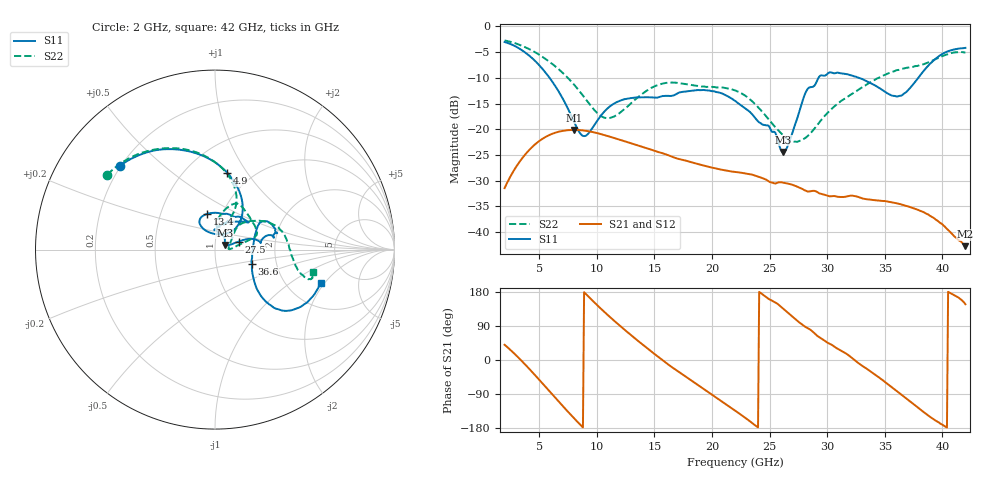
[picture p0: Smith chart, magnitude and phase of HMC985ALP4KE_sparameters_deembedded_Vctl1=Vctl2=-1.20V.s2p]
!s2p File: Measurements: S11, S21, S12, S22
# GHz S dB R 50.0
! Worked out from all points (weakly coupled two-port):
!   401 points, 2 GHz to 42 GHz, reference 50 ohm
!   highest |S21| = -20.11 dB at 8 GHz (marker M1); lowest = -42.7 dB at 42 GHz (marker M2)
!   lowest |S11| = -24.4 dB at 26.2 GHz (marker M3), VSWR 1.13, Z = 55.7 + j2.87 ohm
!   |S11| at or under -10 dB: 5.908 GHz to 29.25 GHz (23.34 GHz wide, 133 % of centre); 32.76 GHz to 37.9 GHz (5.142 GHz wide, 14.6 % of centre)
!   |S22| runs from -22.4 to -2.7 dB; largest |S21 - S12| = 0.00014
!   S11 on the Smith chart (normalised r, x): 2 GHz: 0.20, +0.37; 4.9 GHz: 0.77, +0.81; 13.4 GHz: 0.85, +0.35; 27.5 GHz: 1.30, +0.12; 36.6 GHz: 1.49, -0.25; 42 GHz: 3.03, -1.85
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2  -3.01 138.6  -31.43 40.1  -31.43 40.1  -2.72 145.2
3.4  -4.46 111.1  -26.00 0.2  -26.00 0.2  -3.66 122.3
4.9  -7.28 80.8  -22.44 -48.7  -22.45 -48.7  -5.34 98.8
6.2  -10.92 57.1  -20.81 -93.0  -20.82 -93.0  -7.39 80.8
8  -18.39 51.2  -20.11 -152.8  -20.11 -152.8  -11.23 64.7
8.7  -21.14 73.6  -20.19 -174.9  -20.19 -174.9  -13.15 63.4
10.9  -16.00 120.8  -21.27 120.2  -21.27 120.1  -17.82 81.9
13.4  -13.81 102.5  -23.01 54.9  -23.02 54.9  -14.09 80.9
15.4  -13.73 75.7  -24.45 7.0  -24.45 7.0  -11.30 68.5
18.9  -12.38 40.0  -26.81 -68.6  -26.82 -68.6  -11.60 41.8
22  -14.45 55.3  -28.27 -133.3  -28.28 -133.3  -12.43 18.4
24.9  -19.28 88.1  -30.06 161.6  -30.07 161.5  -18.01 10.1
26.2  -24.41 25.2  -30.37 134.7  -30.38 134.7  -21.22 2.3
27.5  -17.14 18.7  -31.25 101.3  -31.24 101.2  -22.33 6.6
28.2  -12.53 13.3  -32.02 85.7  -32.04 85.7  -21.52 17.4
28.7  -11.76 8.6  -31.98 76.0  -31.98 76.1  -20.37 25.3
31  -9.01 19.6  -33.13 28.2  -33.15 28.2  -14.84 45.4
33.3  -10.49 31.0  -33.55 -20.3  -33.56 -20.4  -11.49 36.8
35.4  -13.19 10.2  -34.11 -66.9  -34.12 -66.9  -9.05 23.3
36.6  -13.17 -21.1  -34.71 -95.0  -34.73 -95.2  -8.21 14.2
39.6  -5.96 -42.3  -37.81 -163.4  -37.85 -163.4  -6.17 -15.1
42  -4.16 -17.7  -42.72 147.1  -42.69 146.9  -5.04 -13.1
